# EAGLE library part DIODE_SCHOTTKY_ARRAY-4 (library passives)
Array of 4 Schottky Diodes Example part: RB521ZS8A30TE61CT-ND
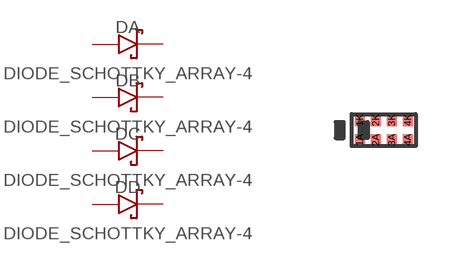
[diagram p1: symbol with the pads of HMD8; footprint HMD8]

Designator prefix D; gates A=DIODE_SCHOTTKY B=DIODE_SCHOTTKY C=DIODE_SCHOTTKY D=DIODE_SCHOTTKY

## DIODE_SCHOTTKY_ARRAY-4HMD8 (DIGIKEY: RB521ZS8A30TE61CT-ND; MANUFACTURER: Rohm Semiconductor; MPN: RB521ZS8A30TE61)  [HMD8]
1A  A:ANODE
1K  A:CATHODE
2A  B:ANODE
2K  B:CATHODE
3A  C:ANODE
3K  C:CATHODE
4A  D:ANODE
4K  D:CATHODE

## Footprint HMD8 (pad centres in mm)
HMD8 Possibly ROHM-specific pacakge Drawn from http://rohmfs.rohm.com/en/products/databook/datasheet/discrete/diode/schottky_barrier/rb521zs8a30.pdf DigiKey RB521ZS8A30TE61CT-ND
smd 0.25 x 0.3: 1A -0.6,-0.25; 1K -0.6,0.25; 2A -0.2,-0.25; 2K -0.2,0.25; 3A 0.2,-0.25; 3K 0.2,0.25; 4A 0.6,-0.25; 4K 0.6,0.25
